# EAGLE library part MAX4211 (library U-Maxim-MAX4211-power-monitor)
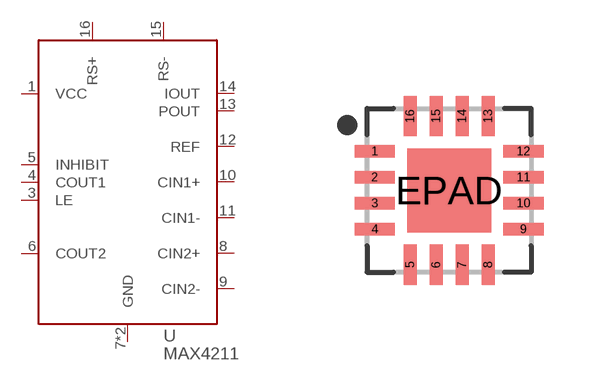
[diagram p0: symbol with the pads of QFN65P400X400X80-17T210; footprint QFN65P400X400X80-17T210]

Designator prefix U

## MAX4211  [QFN65P400X400X80-17T210]
1  VCC  pwr
3  LE  in
4  COUT1  oc
5  INHIBIT  in
6  COUT2  oc
7  GND  pwr
8  CIN2+  in
9  CIN2-  in
10  CIN1+  in
11  CIN1-  in
12  REF  out
13  POUT  out
14  IOUT  out
15  RS-  pas
16  RS+  pas
EPAD  GND  pwr

## Footprint QFN65P400X400X80-17T210 (pad centres in mm)
16-QFN, 0.65 mm pitch, 4.00 X 4.00 X 0.80 mm body, 2.10 X 2.10 mm thermal pad 16-pin QFN package with 0.65 mm pitch with body size 4.00 X 4.00 X 0.80 mm and thermal pad size 2.10 X 2.10 mm
smd 1.01 x 0.32: 1 -1.86,0.975; 2 -1.86,0.325; 3 -1.86,-0.325; 4 -1.86,-0.975; 9 1.86,-0.975; 10 1.86,-0.325; 11 1.86,0.325; 12 1.86,0.975
smd 0.32 x 1.01: 5 -0.975,-1.86; 6 -0.325,-1.86; 7 0.325,-1.86; 8 0.975,-1.86; 13 0.975,1.86; 14 0.325,1.86; 15 -0.325,1.86; 16 -0.975,1.86
smd 2.1 x 2.1: EPAD 0,0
